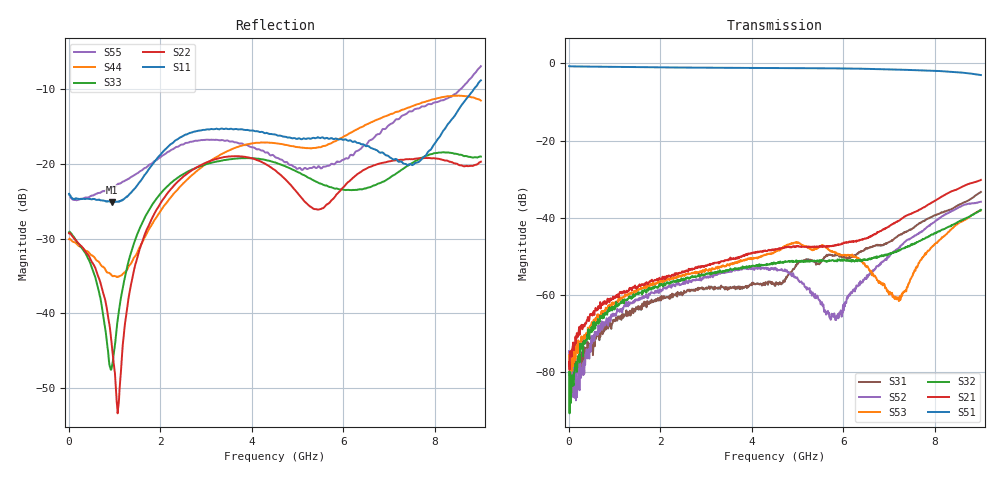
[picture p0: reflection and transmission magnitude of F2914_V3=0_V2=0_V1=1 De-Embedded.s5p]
! Integrated Device Technology
! Corporate Headquarters
! 6024 Silver Creek Valley Road
! San Jose, CA 95138  USA
! Phone:  1-408-284-8200
! Toll Free:  1-800-223-1366
! Webpage:  http://www.idt.com/
! Timing and RF Division
! 515 Groton Road, Suite 102
! Westford, MA 01886-6024
! Device:  F2914
! Description: High Reliability SP4T RF Switch
! Frequency:  0.05 -  8.GHz
! Package:  4x4 mm Thin QFN Plastic Package: 24 pin
! Ports:  5 RF,  5 DC
!  Pin  1  = GND
!  Pin  2  = GND
!  Pin  3  = GND
!  Pin  4  = GND
!  Pin  5  = RF4  =  Port 4
!  Pin  6  = GND
!  Pin  7  = GND
!  Pin  8  = RF3  =  Port 3
!  Pin  9  = GND
!  Pin 10  = GND
!  Pin 11  = RF2  =  Port 2
!  Pin 12  = GND
!  Pin 13  = GND
!  Pin 14  = RF1  =  Port 1
!  Pin 15  = GND
!  Pin 16  = Vcc
!  Pin 17  = V1
!  Pin 18  = V2
!  Pin 19  = V3
!  Pin 20  = VSSext
!  Pin 21  = GND
!  Pin 22  = RFC  =  Port 5
!  Pin 23  = GND
!  Pin 24  = GND
! Voltage:  VDD  =  +3.30 Volts
!  VSSEXT =  0.00 Volts
! Current:  IDD  = 325  uA
! State:  RF1 Selected
! V1:  Logic HIGH
! V2:  Logic LOW
! V3:  Logic LOW
! Data:  The device was measured on the F291x evaluation board which has
!  individual transmission lines to the RF pins.  Data was collected
!  using a calibrated network analyzer.  The input lines were
!  modeled using Automatic Fixture Removal (AFR) from Keysight.
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# Hz S  dB  R 50
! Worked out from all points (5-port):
!   900 points, 10 MHz to 9 GHz, reference 50 ohm
!   strongest paths, dB at 10 MHz, 2.26 GHz, 4.51 GHz, 6.76 GHz, 9 GHz:
!     S51: -0.8, -1.1, -1.2, -1.5, -3.1
!     S21: -77.3, -54.9, -48.3, -43.7, -30.2
!     S32: -79.8, -56.6, -51.8, -50.1, -37.9
!     S53: -75.6, -55.7, -48.8, -56.5, -38.1
!     S52: -74.5, -57.6, -52.9, -52.6, -35.8
!     S31: -77.5, -59.6, -57.7, -47.1, -33.3
!   lowest |S11| = -25.2 dB at 940 MHz (marker M1), VSWR 1.12, Z = 55.8 - j0.22 ohm
!   |S11| at or under -10 dB: start of sweep to 8.852 GHz
